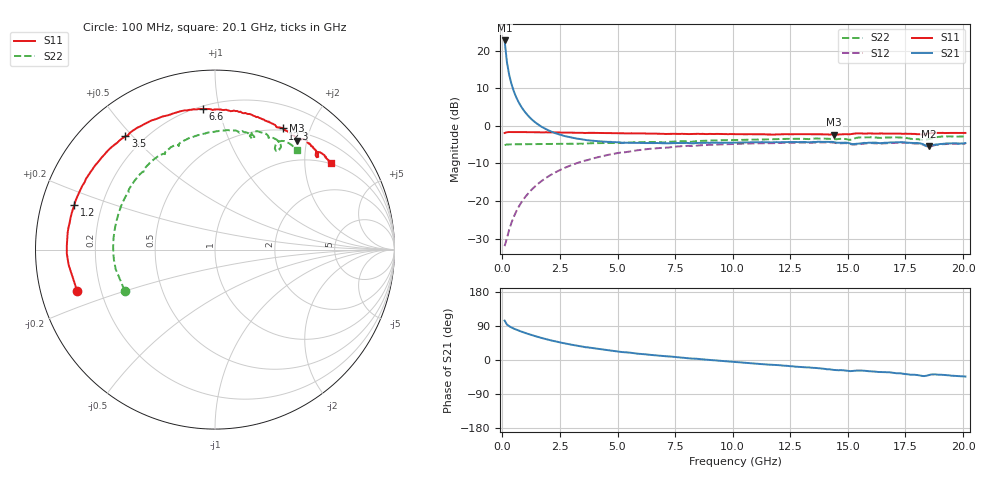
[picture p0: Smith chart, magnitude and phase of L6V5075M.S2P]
!  Infineon Technologies AG
! BFR380L3 , PF131585-7, No.6, Th 09.10.01, soldered on pcb-board, measured with PP GSG850
!  Vce=0.5 V,  Ic=75.0 mA
! Common Emitter S-Parameters:  15. November 2001
#  GHz  S  MA  R  50
! f  S11  S21  S12  S22
! GHz  Mag  Ang  Mag  Ang  Mag  Ang  Mag  Ang
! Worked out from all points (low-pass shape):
!   201 points, 100 MHz to 20.1 GHz, reference 50 ohm
!   highest |S21| = 22.70 dB at 100 MHz (marker M1); lowest = -5.4 dB at 18.5 GHz (marker M2)
!   |S21| within 3 dB of the highest: start of sweep to 152.1 MHz
!   lowest |S11| = -2.4 dB at 14.4 GHz (marker M3), VSWR 7.33, Z = 31.8 + j91.4 ohm
!   |S11| at or under -10 dB: nowhere
!   |S22| runs from -5.1 to -2.8 dB; largest |S21 - S12| = 14
!   S11 on the Smith chart (normalised r, x): 100 MHz: 0.11, -0.15; 1.2 GHz: 0.10, +0.15; 3.5 GHz: 0.13, +0.48; 6.6 GHz: 0.22, +0.89; 12.3 GHz: 0.48, +1.60; 20.1 GHz: 0.99, +2.68
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0.1  0.8018 -163.2  13.64 104.0  0.02507 41.0  0.5529 -155.6
0.2  0.8198 -174.0  7.029 93.7  0.03183 50.9  0.5641 -169.0
0.3  0.8258 -178.4  4.734 89.2  0.04178 57.8  0.5659 -174.3
0.4  0.8258 178.3  3.576 85.7  0.05152 61.5  0.5668 -177.4
0.5  0.8253 175.7  2.876 82.8  0.06165 64.4  0.5673 -179.7
0.6  0.8263 173.5  2.411 80.3  0.07214 65.5  0.5678 178.5
0.7  0.8256 171.5  2.084 77.8  0.0824 66.4  0.568 176.9
0.9  0.824 167.7  1.652 73.4  0.1034 66.7  0.5688 174.1
1.2  0.8215 162.5  1.285 67.3  0.1341 65.8  0.5697 170.4
1.5  0.8213 157.5  1.07 61.7  0.1643 64.1  0.5703 167.1
2  0.8185 149.7  0.8702 53.4  0.2125 60.1  0.5724 161.8
3.5  0.8052 128.4  0.6569 35.2  0.3395 46.4  0.5772 147.1
6.6  0.7865 95.0  0.5886 12.6  0.4995 20.6  0.6091 120.2
6.8  0.7842 93.1  0.5888 11.4  0.5063 19.1  0.6068 118.5
10.1  0.7743 71.1  0.5955 -5.2  0.5735 -1.4  0.647 96.9
12.3  0.7734 60.8  0.6054 -15.2  0.5952 -13.1  0.6699 83.8
13.5  0.7744 55.8  0.6108 -20.8  0.5985 -19.0  0.6716 77.6
14.4  0.76 53.1  0.6043 -26.3  0.596 -24.9  0.6618 72.9
16.8  0.7891 45.4  0.5995 -32.4  0.5881 -31.7  0.7008 62.8
18.2  0.7653 42.2  0.5782 -41.8  0.5706 -41.2  0.6516 57.3
18.5  0.7896 43.6  0.536 -40.2  0.5293 -39.1  0.664 59.7
20.1  0.8037 36.8  0.5891 -43.6  0.5783 -43.1  0.7208 50.6
